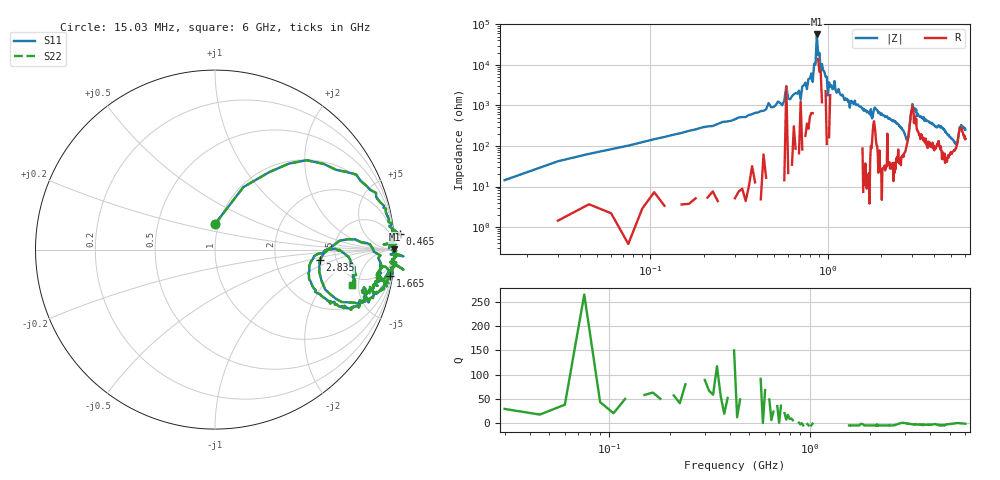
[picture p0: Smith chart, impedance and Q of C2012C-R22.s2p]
!	Network	Analyzer	HP8753E.07.74:	Oct	30	2002	Serial	No.	JP38451487
!	Hewlett-Packard
!	7	Sep	2009	12:18:27
!	Frequency	S11	S21	S12	S22
#	HZ	S	RI	R	50
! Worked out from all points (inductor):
!   400 points, 15.03 MHz to 6 GHz, reference 50 ohm
!   read as one part in series: L = 219 nH near 45.03 MHz
!   highest |Z| = 56.2 kohm at 870 MHz (marker M1)
!   self-resonance near 885 MHz
!   S11 on the Smith chart (normalised r, x): 15.03 MHz: 0.96, +0.29; 465 MHz: -8, +21; 1.665 GHz: 1, -13; 2.835 GHz: 3.70, -0.66; 6 GHz: 3.95, -4.18
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1.502992e7  0.00192 0.145  0.998 -0.145  0.998 -0.145  0.00192 0.145
3.002985e7  0.158 0.348  0.842 -0.348  0.842 -0.348  0.158 0.348
9.002955e7  0.607 0.477  0.393 -0.477  0.393 -0.477  0.607 0.477
4.650277e8  1.03 0.0851  -0.0292 -0.0851  -0.0292 -0.0851  1.03 0.0851
5.550272e8  0.992 0.0982  0.00772 -0.0982  0.00772 -0.0982  0.992 0.0982
5.850271e8  0.969 0.00714  0.0313 -0.00714  0.0313 -0.00714  0.969 0.00714
7.050265e8  0.94 0.0286  0.0603 -0.0286  0.0603 -0.0286  0.94 0.0286
8.250259e8  0.995 0.0257  0.0051 -0.0257  0.0051 -0.0257  0.995 0.0257
8.550257e8  0.99 0.000488  0.00967 -0.000488  0.00967 -0.000488  0.99 0.000488
8.700256e8  1 0.00177  -0.00018 -0.00177  -0.00018 -0.00177  1 0.00177
9.150254e8  0.986 -0.0025  0.014 0.0025  0.014 0.0025  0.986 -0.0025
9.90025e8  0.999 -0.0197  0.000824 0.0197  0.000824 0.0197  0.999 -0.0197
1.005025e9  1.05 -0.0376  -0.0461 0.0376  -0.0461 0.0376  1.05 -0.0376
1.020025e9  0.998 -0.0269  0.00192 0.0269  0.00192 0.0269  0.998 -0.0269
1.335023e9  1.05 -0.111  -0.045 0.111  -0.045 0.111  1.05 -0.111
1.665022e9  0.976 -0.145  0.0235 0.145  0.0235 0.145  0.976 -0.145
2.01002e9  0.97 -0.154  0.0304 0.154  0.0304 0.154  0.97 -0.154
2.835016e9  0.583 -0.0584  0.417 0.0584  0.417 0.0584  0.583 -0.0584
3.015015e9  0.922 -0.0324  0.0782 0.0324  0.0782 0.0324  0.922 -0.0324
4.00501e9  0.86 -0.243  0.14 0.243  0.14 0.243  0.86 -0.243
5.010005e9  0.646 -0.289  0.354 0.289  0.354 0.289  0.646 -0.289
6e9  0.764 -0.199  0.236 0.199  0.236 0.199  0.764 -0.199
